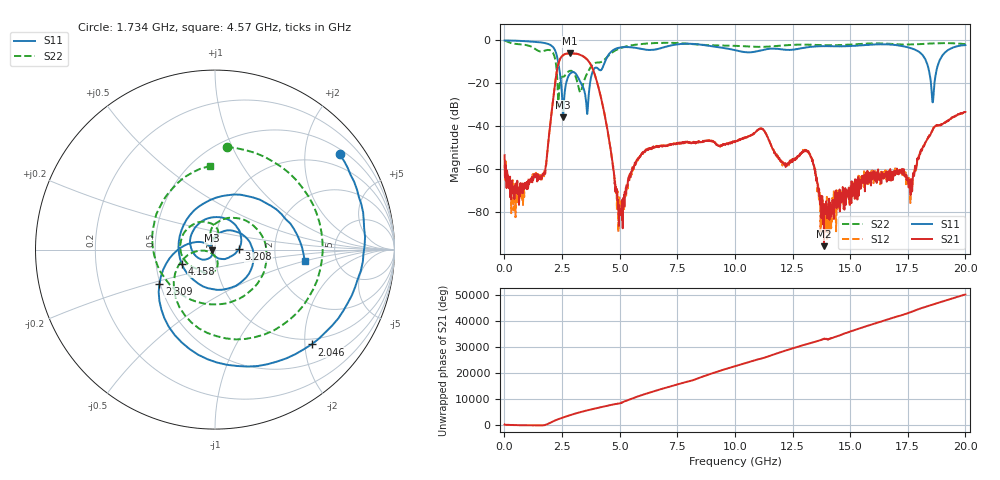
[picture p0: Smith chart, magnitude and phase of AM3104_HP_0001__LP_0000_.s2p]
!Created with skrf (http://scikit-rf.org).
# Hz S RI R 50.0
!freq ReS11 ImS11 ReS21 ImS21 ReS12 ImS12 ReS22 ImS22
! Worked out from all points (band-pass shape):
!   1601 points, 10 MHz to 20 GHz, reference 50 ohm
!   highest |S21| = -6.00 dB at 2.846 GHz (marker M1); lowest = -96.0 dB at 13.87 GHz (marker M2)
!   |S21| within 3 dB of the highest: 2.402 GHz to 3.601 GHz (1.199 GHz wide, 40 % of centre)
!   lowest |S11| = -35.8 dB at 2.546 GHz (marker M3), VSWR 1.03, Z = 48.4 - j0.363 ohm
!   |S11| at or under -10 dB: 2.331 GHz to 4.362 GHz (2.031 GHz wide, 60.7 % of centre); 18.31 GHz to 18.86 GHz (549 MHz wide, 2.95 % of centre)
!   |S22| runs from -30.9 to -0.2 dB; largest |S21 - S12| = 0.004
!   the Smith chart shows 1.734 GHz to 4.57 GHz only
!   S11 on the Smith chart (normalised r, x): 1.734 GHz: 0.63, +2.83; 2.046 GHz: 0.88, -2.14; 2.309 GHz: 0.50, -0.22; 3.208 GHz: 1.31, +0.01; 4.158 GHz: 0.68, -0.11; 4.57 GHz: 2.94, -0.49
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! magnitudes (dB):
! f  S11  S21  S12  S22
! 10 MHz  0.0  -53.5  -58.0  -0.2
! 522.2 MHz  -0.2  -66.5  -71.1  -1.7
! 1.734 GHz  -1.2  -61.9  -62.7  -4.8
! 2.046 GHz  -2.5  -33.7  -33.8  -5.0
! 2.309 GHz  -8.8  -12.4  -12.4  -21.1
! 2.546 GHz  -35.8  -6.9  -6.9  -16.9
! 2.846 GHz  -15.6  -6.0  -6.0  -14.2
! 3.208 GHz  -17.5  -6.4  -6.4  -21.4
! 3.346 GHz  -20.5  -7.0  -7.0  -23.0
! 4.158 GHz  -13.9  -25.2  -25.1  -10.2
! 4.57 GHz  -6.0  -48.5  -48.1  -6.6
! 5.032 GHz  -3.3  -81.5  -78.4  -3.6
! 5.72 GHz  -3.5  -56.8  -57.2  -2.0
! 6.682 GHz  -3.9  -49.8  -49.4  -1.2
! 10.01 GHz  -4.5  -47.3  -47.3  -2.5
! 13.34 GHz  -2.9  -55.3  -56.0  -2.1
! 13.87 GHz  -2.7  -96.0  -75.7  -2.2
! 16.68 GHz  -1.9  -63.2  -64.3  -1.5
! 17.61 GHz  -3.5  -70.3  -75.9  -1.9
! 18.59 GHz  -28.8  -41.7  -41.6  -1.4
! 19.01 GHz  -6.8  -39.0  -39.0  -1.2
! 20 GHz  -2.2  -33.4  -33.4  -1.7
